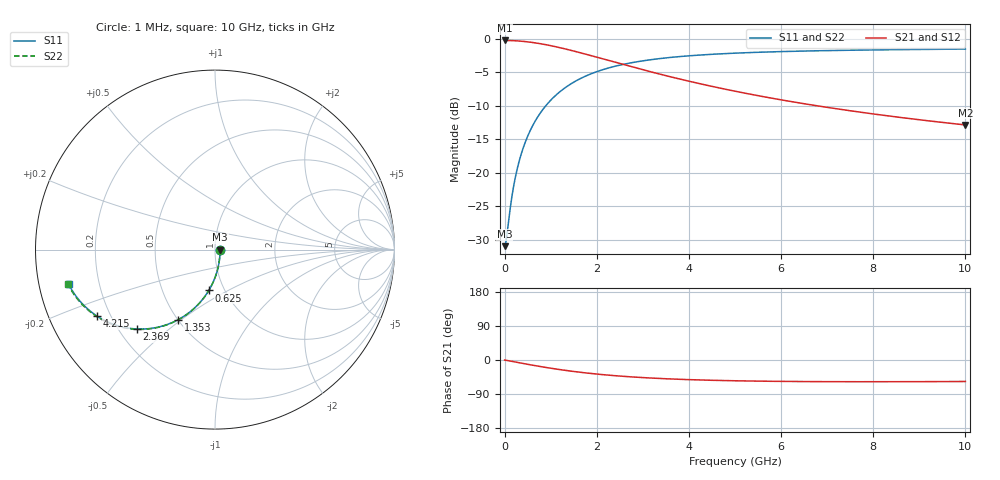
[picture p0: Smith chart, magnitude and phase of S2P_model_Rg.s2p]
! Created Fri Oct 06 12:26:37 2017
# hz S ma R 50
! 2 Port Network Data from SP1.SP block
! freq  magS11  angS11  magS21  angS21  magS12  angS12  magS22  angS22
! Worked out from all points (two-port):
!   10000 points, 1 MHz to 10 GHz, reference 50 ohm
!   highest |S21| = -0.25 dB at 1 MHz (marker M1); lowest = -12.8 dB at 10 GHz (marker M2)
!   |S21| within 3 dB of the highest: start of sweep to 2.268 GHz
!   lowest |S11| = -30.9 dB at 1 MHz (marker M3), VSWR 1.06, Z = 52.9 - j0.0415 ohm
!   |S11| at or under -10 dB: start of sweep to 893 MHz
!   |S22| runs from -30.9 to -1.5 dB; largest |S21 - S12| = 0
!   S11 on the Smith chart (normalised r, x): 1 MHz: 1.06, -0.00; 625 MHz: 0.84, -0.41; 1.353 GHz: 0.50, -0.49; 2.369 GHz: 0.27, -0.39; 4.215 GHz: 0.15, -0.26; 10 GHz: 0.09, -0.12
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1000000  0.02845 -0.8  0.9716 -0.0  0.9716 -0.0  0.02845 -0.8
2.5e7  0.03 -19.1  0.9715 -0.6  0.9715 -0.6  0.03001 -19.2
5e7  0.0342 -35.0  0.9713 -1.2  0.9713 -1.2  0.03425 -35.1
1.34e8  0.05818 -64.1  0.9698 -3.1  0.9698 -3.1  0.05839 -64.3
1.83e8  0.07482 -72.3  0.9684 -4.2  0.9684 -4.2  0.07512 -72.4
2.81e8  0.1095 -82.1  0.9641 -6.5  0.9641 -6.5  0.11 -82.2
3.52e8  0.135 -86.8  0.96 -8.1  0.96 -8.1  0.1356 -86.9
4.33e8  0.1638 -91.0  0.9542 -9.9  0.9542 -9.9  0.1645 -91.1
6.25e8  0.2302 -98.6  0.9365 -14.1  0.9365 -14.1  0.2313 -98.6
7.75e8  0.2795 -103.4  0.9192 -17.2  0.9192 -17.2  0.2808 -103.4
9.45e8  0.3318 -108.2  0.8967 -20.6  0.8967 -20.6  0.3334 -108.2
1.137e9  0.3862 -112.9  0.8684 -24.2  0.8684 -24.2  0.388 -113.0
1.353e9  0.4411 -117.7  0.8343 -27.9  0.8343 -27.9  0.4432 -117.8
1.668e9  0.5096 -123.9  0.7828 -32.8  0.7828 -32.8  0.512 -123.9
2.369e9  0.6205 -134.5  0.6728 -41.2  0.6728 -41.2  0.6234 -134.6
2.836e9  0.6705 -139.9  0.6084 -45.2  0.6084 -45.2  0.6737 -139.9
3.334e9  0.7096 -144.6  0.5489 -48.6  0.5489 -48.6  0.713 -144.6
4.215e9  0.7555 -150.8  0.4644 -52.6  0.4644 -52.6  0.7591 -150.8
5.001e9  0.7813 -154.8  0.4067 -54.8  0.4067 -54.8  0.785 -154.8
6.667e9  0.8124 -160.6  0.3211 -57.0  0.3211 -57.0  0.8162 -160.6
8.334e9  0.8285 -164.2  0.2659 -57.3  0.2659 -57.3  0.8324 -164.2
1e10  0.8379 -166.7  0.2279 -56.7  0.2279 -56.7  0.8419 -166.7
